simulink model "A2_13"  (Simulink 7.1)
settings: Solver=ode1  StartTime=0.0  StopTime=100.0  FixedStep=2e-1  RelTol=1e-3

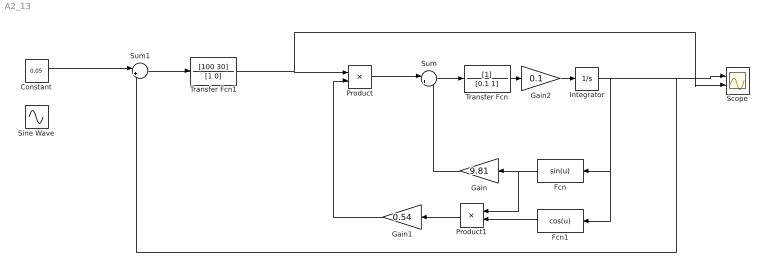
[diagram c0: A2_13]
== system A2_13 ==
  Constant : Constant  Value=0.05  OutDataType=sfix(16)  OutScaling=2^0
  Fcn : Fcn  Orientation=left  Expr=sin(u)
  Fcn1 : Fcn  Orientation=left  Expr=cos(u)
  Gain : Gain  Orientation=left  Gain=9.81  ParameterDataType=sfix(16)  ParameterScaling=2^0  OutDataType=sfix(16)  OutScaling=2^0
  Gain1 : Gain  Orientation=left  Gain=0.54  ParameterDataType=sfix(16)  ParameterScaling=2^0  OutDataType=sfix(16)  OutScaling=2^0
  Gain2 : Gain  Gain=0.1  ParameterDataType=sfix(16)  ParameterScaling=2^0  OutDataType=sfix(16)  OutScaling=2^0
  Integrator : Integrator  InitialCondition=0.01
  Product : Product  OutDataType=sfix(16)  OutScaling=2^0
  Product1 : Product  Orientation=left  OutDataType=sfix(16)  OutScaling=2^0
  Scope : Scope  NumInputPorts=2
  Sine Wave : Sin  Amplitude=0.5  Bias=0.8  SampleTime=0
  Sum : Sum  Inputs=|+-  OutDataType=sfix(16)  OutScaling=2^0
  Sum1 : Sum  Inputs=|+-  OutDataType=sfix(16)  OutScaling=2^0
  Transfer Fcn : TransferFcn  Denominator=[0.1 1]
  Transfer Fcn1 : TransferFcn  Numerator=[100 30]  Denominator=[1 0]
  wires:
  Transfer Fcn/1 -> Gain2/1
  Integrator/1 -> Fcn/1, Fcn1/1, Scope/1, Sum1/2
  Sum/1 -> Transfer Fcn/1
  Product/1 -> Sum/1
  Fcn1/1 -> Product1/2
  Fcn/1 -> Product1/1, Gain/1
  Gain/1 -> Sum/2
  Product1/1 -> Gain1/1
  Gain1/1 -> Product/2
  Transfer Fcn1/1 -> Product/1, Scope/2
  Sum1/1 -> Transfer Fcn1/1
  Gain2/1 -> Integrator/1
  Constant/1 -> Sum1/1
